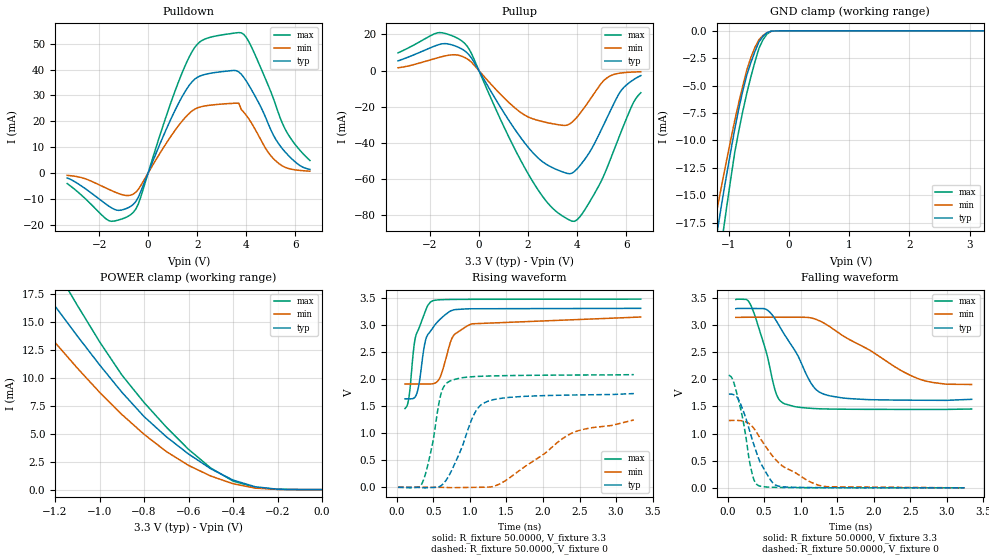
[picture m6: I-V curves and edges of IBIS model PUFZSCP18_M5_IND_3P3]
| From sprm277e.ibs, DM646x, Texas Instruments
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|   Model Cell PUFZSCP18_M5_IND_3P3
[Model]   PUFZSCP18_M5_IND_3P3
Model_type   I/O
Polarity   Non-Inverting
Enable   Active-Low
Vinl =  0.8V
Vinh =  2V
Cref =  10.0000pF
Rref =  50.0000
Vref =  1.5V
Vmeas =  1.65
C_comp   1.716149p   1.667102p   1.755986p
[Model Spec]
Vinl   0.8V   0.8V   0.8V
Vinh   2V   2V   2V
[Temperature Range]   25   125   -40
[Voltage Range]   3.3   3.14   3.47
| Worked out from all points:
|   slope of the pulldown table from 0 to 0.495 V, typ, clamps not added: 42.9 ohm
|   slope of the pullup table from 0 to 0.495 V, typ, clamps not added: 42.8 ohm
|   GND clamp passes 1 mA (typ) near -0.50 V on its own axis
|   POWER clamp passes 1 mA (typ) near -0.41 V on its own axis
|   rising waveform, R_fixture 50.0000, V_fixture 3.3: 20-80 % time 195ps typ, 245ps min, 157ps max; typ from 1.63 V to 3.3 V
|   rising waveform, R_fixture 50.0000, V_fixture 0: 20-80 % time 310ps typ, 768ps min, 168ps max; typ from 0 V to 1.73 V
|   falling waveform, R_fixture 50.0000, V_fixture 3.3: 20-80 % time 411ps typ, 908ps min, 239ps max; typ from 3.3 V to 1.63 V
|   falling waveform, R_fixture 50.0000, V_fixture 0: 20-80 % time 275ps typ, 552ps min, 170ps max; typ from 1.73 V to 0 V
[POWER_clamp]
|   voltage   I(typ)   I(min)   I(max)
-3.3V     86.16mA    64.93mA    104.3mA
-1.367V   21.2mA     17.18mA    25.65mA
-1.233V   17.37mA    13.97mA    21.04mA
-1.133V   14.65mA    11.65mA    17.64mA
-1.1V     13.76mA    10.89mA    16.51mA
-900mV    8.728mA    6.735mA    10.27mA
-800mV    6.541mA    4.954mA    7.803mA
-700mV    4.737mA    3.409mA    5.6mA
-500mV    1.861mA    1.215mA    1.93mA
-400mV    851.5uA    523.4uA    761.4uA
-300mV    252.3uA    131.7uA    194.1uA
0V        112.3nA    202.2nA    235.3nA
[Pulldown]
|   voltage   I(typ)   I(min)   I(max)
-3.3V     -1.944mA   -917.2uA   -4.091mA
-1.6V     -12.83mA   -6.342mA   -18.45mA
-700mV    -12.84mA   -8.548mA   -16.04mA
-400mV    -9.372mA   -6.338mA   -12.02mA
900mV     20.28mA    13.8mA     26.48mA
1.8V      35.39mA    24.06mA    47.09mA
2.3V      38.1mA     25.92mA    51.77mA
3.7V      39.1mA     27mA       54.34mA
4.2V      32.49mA    19.57mA    49.06mA
5.2V      13.12mA    4.726mA    26.38mA
5.7V      6.992mA    1.816mA    15.11mA
6.6V      1.393mA    706.9uA    4.852mA
[Pullup]
|   voltage   I(typ)   I(min)   I(max)
-3.3V     5.394mA    1.595mA    9.842mA
-1.7V     14.1mA     7.032mA    20.86mA
-600mV    11.14mA    7.393mA    15.31mA
1.3V      -29.12mA   -18.59mA   -38.9mA
2.2V      -45.34mA   -26.61mA   -61.37mA
3V        -53.59mA   -29.31mA   -75.93mA
3.8V      -56.58mA   -28.42mA   -83.16mA
4.3V      -49.27mA   -20.37mA   -77.23mA
5.2V      -26.7mA    -4.187mA   -54.48mA
5.8V      -10.97mA   -1.281mA   -33.72mA
6.3V      -5.031mA   -754.8uA   -17.64mA
6.6V      -2.731mA   -599.9uA   -12.21mA
[GND_clamp]
|   voltage   I(typ)   I(min)   I(max)
-3.3V     -101.7mA   -78.08mA   -120.7mA
-1.3V     -22.2mA    -19.34mA   -26.65mA
-1.233V   -19.78mA   -17.4mA    -23.95mA
-1.167V   -17.44mA   -15.48mA   -21.27mA
-1.1V     -15.19mA   -13.58mA   -18.61mA
-1.033V   -13.05mA   -11.73mA   -16mA
-900mV    -8.932mA   -8.157mA   -11.06mA
-700mV    -4.017mA   -3.556mA   -5.673mA
-500mV    -1.012mA   -805.8uA   -1.608mA
-366.7mV  -174uA     -171uA     -303.7uA
-166.7mV  -4.976uA   -6.043uA   -6.59uA
3.233V    80.15nA    2.439uA    205.5nA
[Ramp]
| variable   typ   min   max
dV/dt_f  1.0170401/0.41788058n 0.77591599/0.95862958n  1.2188332/0.24032471n
dV/dt_r  1.0440199/0.31185825n  0.7592554/0.78998528n  1.2536284/0.16941246n
R_load = 50
[Rising Waveform]
R_fixture = 50.0000
V_fixture = 3.3
V_fixture_min = 3.14
V_fixture_max = 3.47
|   time   V(typ)   V(min)   V(max)
112.5ps   1.631V     1.904V     1.452V
169ps     1.631V     1.905V     1.68V
258.5ps   1.681V     1.905V     2.782V
306.1ps   1.916V     1.905V     2.941V
392.7ps   2.706V     1.905V     3.253V
490.3ps   2.934V     1.908V     3.439V
593.2ps   3.099V     2.031V     3.458V
773.8ps   3.269V     2.791V     3.464V
1.025ns   3.292V     3.015V     3.467V
3.338ns   3.3V       3.14V      3.47V
[Rising Waveform]
R_fixture = 50.0000
V_fixture = 0
V_fixture_min = 0
V_fixture_max = 0
|   time   V(typ)   V(min)   V(max)
17.55ps   36.66uV    21.26uV    58.27uV
351.8ps   -8.62mV    28.83uV    89.99mV
481.1ps   -4.881mV   -510.9uV   749.1mV
602.9ps   26.29mV    -1.729mV   1.711V
731.4ps   258.8mV    -6.402mV   1.961V
1.063ns   1.358V     -1.585mV   2.041V
1.238ns   1.582V     2.447mV    2.051V
1.5ns     1.653V     133.3mV    2.059V
2.385ns   1.701V     992.4mV    2.07V
3.243ns   1.728V     1.241V     2.077V
[Falling Waveform]
R_fixture = 50.0000
V_fixture = 3.3
V_fixture_min = 3.14
V_fixture_max = 3.47
|   time   V(typ)   V(min)   V(max)
112.5ps   3.3V       3.14V      3.47V
253.7ps   3.305V     3.142V     3.47V
318.7ps   3.304V     3.143V     3.36V
528ps     3.288V     3.143V     2.504V
660.8ps   3.088V     3.143V     1.752V
779.8ps   2.819V     3.142V     1.548V
1.159ns   1.894V     3.124V     1.463V
1.337ns   1.717V     3.02V      1.453V
2.56ns    1.614V     2.036V     1.445V
3.338ns   1.631V     1.904V     1.452V
[Falling Waveform]
R_fixture = 50.0000
V_fixture = 0
V_fixture_min = 0
V_fixture_max = 0
|   time   V(typ)   V(min)   V(max)
17.55ps   1.728V     1.241V     2.077V
79.63ps   1.717V     1.242V     1.959V
166.4ps   1.581V     1.239V     1.522V
225.1ps   1.38V      1.226V     1.14V
328ps     929.3mV    1.146V     307.2mV
368.7ps   756.4mV    1.079V     123.7mV
427.7ps   531.2mV    954.6mV    39.23mV
657.8ps   51.14mV    519.7mV    8.81mV
1.239ns   4.785mV    50.51mV    2.411mV
3.243ns   36.66uV    21.26uV    58.27uV
